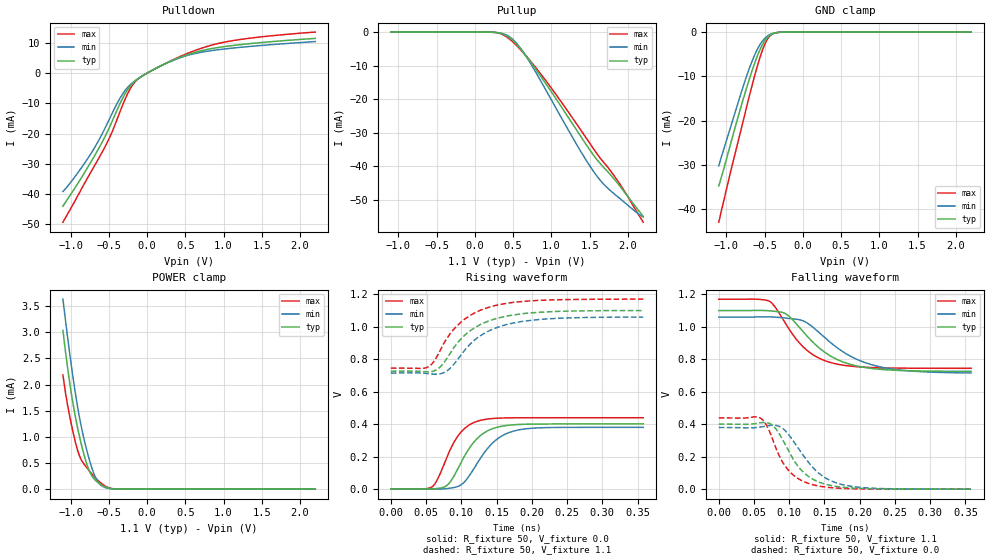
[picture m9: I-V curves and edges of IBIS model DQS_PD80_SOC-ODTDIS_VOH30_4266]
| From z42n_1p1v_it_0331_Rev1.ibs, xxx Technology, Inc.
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| DQS_PD80_SOC-ODTDIS_VOH30_4266
| (80 Ohm Pulldown, SOC ODT disabled setting, VOH=VDDQ/3.0 cal. point, 3200-4266Mbps)
[Model]   DQS_PD80_SOC-ODTDIS_VOH30_4266
Model_type   I/O
Vinl = 123.333mV
Vinh = 243.333mV
Vmeas = 183.333mV
Vref = 0.0mV
Cref = 0.0pF
|   typ   min   max
|C_comp   0.849pF   0.799pF   0.899pF
C_comp_pullup   0.4245pF   0.3995pF   0.4495pF
C_comp_pulldown   0.4245pF   0.3995pF   0.4495pF
| Note: C_comp changes when the ODT circuit is enabled.
[Model Spec]
| Input threshold voltage corners
Vinl   0.1233V   0.1167V   0.1350V
Vinh   0.2433V   0.2367V   0.2550V
| Measurement voltage corners
Vmeas   0.1833V   0.1767V   0.1950V
| Timing spec test load voltage corners
Vref   0.0000V   0.0000V   0.0000V
| Dynamic Overshoot Parameters from LPDDR4 Specification
D_overshoot_ampl_h   0.30   NA   NA
D_overshoot_ampl_l   0.30   NA   NA
D_overshoot_area_h   0.1n   NA   NA
D_overshoot_area_l   0.1n   NA   NA
[Voltage Range]   1.1000V   1.0600V   1.1700V
[Pullup Reference]   1.1000V   1.0600V   1.1700V
| Junction Temperature (Ambient temp is 35C typ 95C min -40C max)
[Temperature Range]   50.0   110.0   -40.0
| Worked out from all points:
|   slope of the pulldown table from 0 to 0.165 V, typ, clamps not added: 73.9 ohm
|   slope of the pullup table from 0 to 0.165 V, typ, clamps not added: 13 kohm
|   GND clamp passes 1 mA (typ) near -0.45 V on its own axis
|   POWER clamp passes 1 mA (typ) near -0.88 V on its own axis
|   rising waveform, R_fixture 50, V_fixture 0.0: 20-80 % time 35.2ps typ, 39.3ps min, 30.4ps max; typ from 0.001 V to 0.401 V
|   falling waveform, R_fixture 50, V_fixture 1.1: 20-80 % time 58.3ps typ, 68.9ps min, 47.4ps max; typ from 1.1 V to 0.726 V
|   rising waveform, R_fixture 50, V_fixture 1.1: 20-80 % time 53.9ps typ, 55.4ps min, 51.8ps max; typ from 0.726 V to 1.1 V
|   falling waveform, R_fixture 50, V_fixture 0.0: 20-80 % time 38ps typ, 44.2ps min, 33.1ps max; typ from 0.401 V to 0.001 V
[Pulldown]
|   Voltage   I(typ)   I(min)   I(max)
-1.1V     -44.04mA   -39.15mA   -49.32mA
-918.5mV  -37.06mA   -33.44mA   -41.18mA
-717.2mV  -28.69mA   -25.98mA   -32mA
-499.4mV  -18.39mA   -15.62mA   -21.85mA
-311.3mV  -7.943mA   -6.615mA   -10.1mA
-199.1mV  -3.704mA   -3.385mA   -4.326mA
-93.5mV   -1.474mA   -1.439mA   -1.485mA
388.3mV   4.785mA    4.676mA    4.965mA
596.2mV   6.626mA    6.292mA    7.181mA
889.9mV   8.305mA    7.596mA    9.551mA
1.375V    9.822mA    8.882mA    11.64mA
2.2V      11.48mA    10.44mA    13.57mA
[GND Clamp]
|   Voltage   I(typ)   I(min)   I(max)
-1.1V     -34.74mA   -30.21mA   -42.91mA
-1.05V    -31.86mA   -27.33mA   -39.27mA
-938.3mV  -24.81mA   -21.07mA   -31.08mA
-786.5mV  -15.53mA   -12.6mA    -20.49mA
-667.7mV  -8.907mA   -6.722mA   -12.29mA
-591.8mV  -5.255mA   -3.789mA   -7.492mA
-519.2mV  -2.564mA   -1.833mA   -3.66mA
-466.4mV  -1.294mA   -942.4uA   -1.691mA
-413.6mV  -563.9uA   -416.3uA   -620.9uA
-350.9mV  -165.7uA   -126.1uA   -147.4uA
-261.8mV  -17.65uA   -15.5uA    -11.07uA
2.2V      0A         0A         0A
[Pullup]
|   Voltage   I(typ)   I(min)   I(max)
-1.1V     6.275uA    9.671uA    2.829uA
226.6mV   -42.09uA   -42.88uA   -42.77uA
338.8mV   -360.6uA   -299.8uA   -496.1uA
434.5mV   -1.386mA   -1.132mA   -1.75mA
550mV     -3.794mA   -3.486mA   -4.131mA
695.2mV   -7.909mA   -8.164mA   -7.815mA
1.009V    -18.16mA   -20.62mA   -17.03mA
1.365V    -30.49mA   -34.9mA    -28.6mA
1.576V    -37.53mA   -42.43mA   -35.7mA
1.688V    -40.51mA   -45.51mA   -39.01mA
1.887V    -45.73mA   -49.52mA   -45.08mA
2.2V      -55.05mA   -55.17mA   -56.74mA
[POWER Clamp]
|   Voltage   I(typ)   I(min)   I(max)
-1.1V     3.033mA    3.633mA    2.184mA
-1.041V   2.345mA    2.929mA    1.625mA
-968mV    1.637mA    2.139mA    1.094mA
-902mV    1.132mA    1.525mA    716.8uA
-845.9mV  780uA      1.103mA    527.5uA
-776.6mV  434.2uA    683.3uA    390.2uA
-710.6mV  232.2uA    359uA      273.1uA
-654.5mV  142.7uA    170.5uA    185.9uA
-591.8mV  77.91uA    64.8uA     105.5uA
-492.8mV  18.87uA    11.58uA    24.07uA
-383.9mV  1.736uA    1.207uA    1.465uA
2.2V      0A         0A         0A
[Ramp]
|   typ   min   max
| 20% - 80%
dV/dt_r   240.17m/35.18p   227.73m/39.33p   263.25m/30.37p
dV/dt_f   224.44m/58.23p   206.40m/68.94p   255.17m/47.47p
| 25% - 75%
|dV/dt_r   200.15m/28.01p   189.78m/31.30p   219.38m/24.16p
|dV/dt_f   187.04m/46.37p   172.00m/54.84p   212.64m/37.72p
R_load = 50
[Rising Waveform]
R_fixture = 50
V_fixture = 0.0
|   Time   V(typ)   V(min)   V(max)
0s        806.6uV    708.8uV    583.1uV
59ps      732.4uV    -243.3uV   15.32mV
67ps      4.234mV    -490.3uV   66.67mV
79ps      20.64mV    2.823mV    190.8mV
95ps      124.2mV    16mV       325.6mV
107ps     221.6mV    56.78mV    381.8mV
125ps     321.6mV    175.6mV    420.8mV
150ps     379.8mV    305mV      436.1mV
181ps     397.7mV    364.1mV    439.1mV
358ps     401.1mV    380.3mV    439.3mV
[Falling Waveform]
R_fixture   = 50
V_fixture   = 1.1
V_fixture_min = 1.06
V_fixture_max = 1.17
|   Time   V(typ)   V(min)   V(max)
0s        1.1V       1.06V      1.17V
73ps      1.098V     1.061V     1.155V
95ps      1.08V      1.054V     1.019V
119ps     973.8mV    1.038V     879.9mV
137ps     890.9mV    985.2mV    819.3mV
158ps     821.8mV    905mV      781.1mV
191ps     764mV      809.8mV    756.3mV
227ps     739.2mV    755.6mV    748mV
272ps     729.3mV    728.1mV    745.4mV
358ps     725.9mV    716mV      744.7mV
[Rising Waveform]
R_fixture   = 50
V_fixture   = 1.1
V_fixture_min = 1.06
V_fixture_max = 1.17
|   Time   V(typ)   V(min)   V(max)
0s        725.5mV    714.2mV    744.7mV
52ps      721.4mV    711.1mV    750.9mV
62ps      728.5mV    707.4mV    791.3mV
75ps      776.9mV    716.5mV    895.2mV
89ps      868.3mV    766.3mV    982.5mV
106ps     951.7mV    861.5mV    1.05V
123ps     1.004V     931.9mV    1.093V
144ps     1.043V     983.7mV    1.126V
209ps     1.088V     1.044V     1.162V
358ps     1.099V     1.059V     1.17V
[Falling Waveform]
R_fixture = 50
V_fixture = 0.0
|   Time   V(typ)   V(min)   V(max)
0s        401.2mV    380.4mV    439.4mV
57ps      408.1mV    381.8mV    442.2mV
74ps      400.8mV    393.6mV    335.7mV
86ps      340.9mV    386.9mV    204.3mV
97ps      253.5mV    348.1mV    126.9mV
113ps     138.6mV    251.5mV    64.66mV
131ps     68.22mV    146.4mV    30.69mV
154ps     28.13mV    63.17mV    12.16mV
187ps     8.459mV    18.8mV     3.552mV
358ps     875.9uV    831.1uV    607uV
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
